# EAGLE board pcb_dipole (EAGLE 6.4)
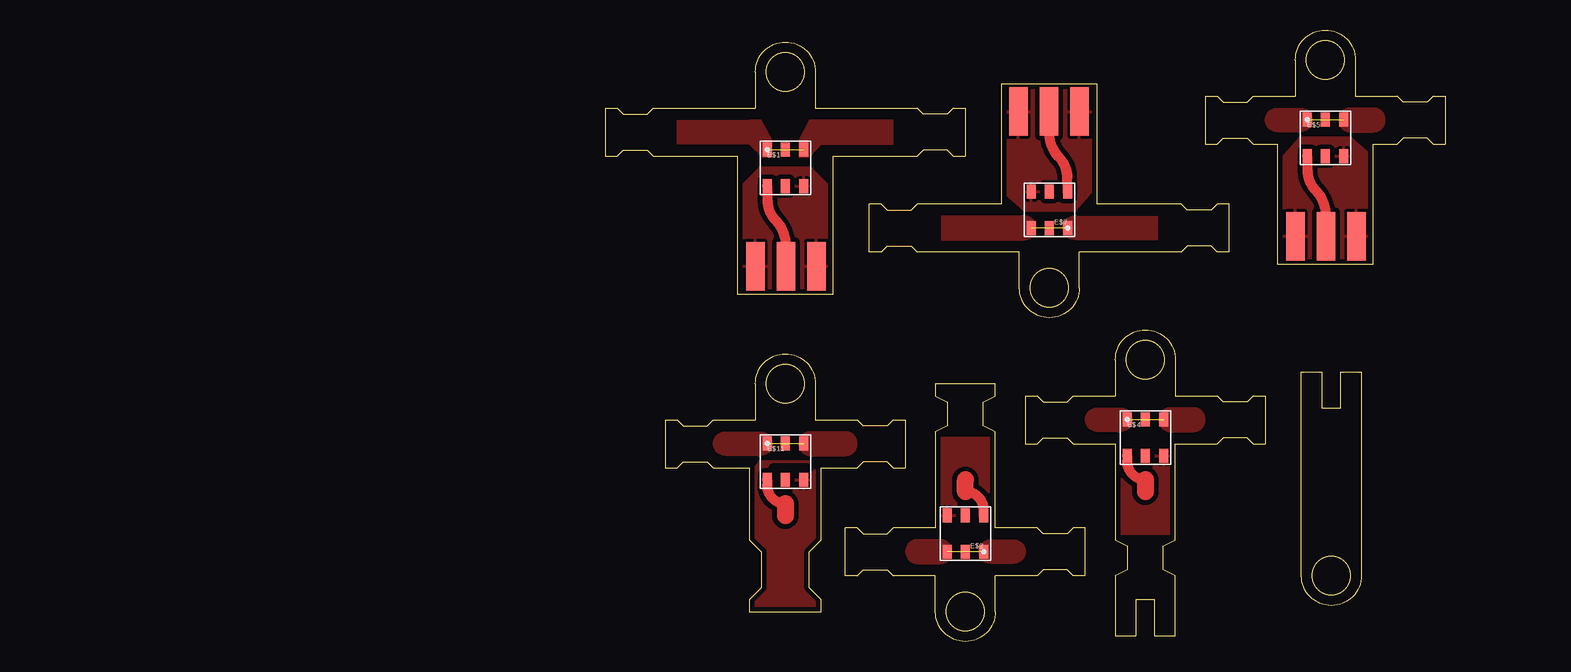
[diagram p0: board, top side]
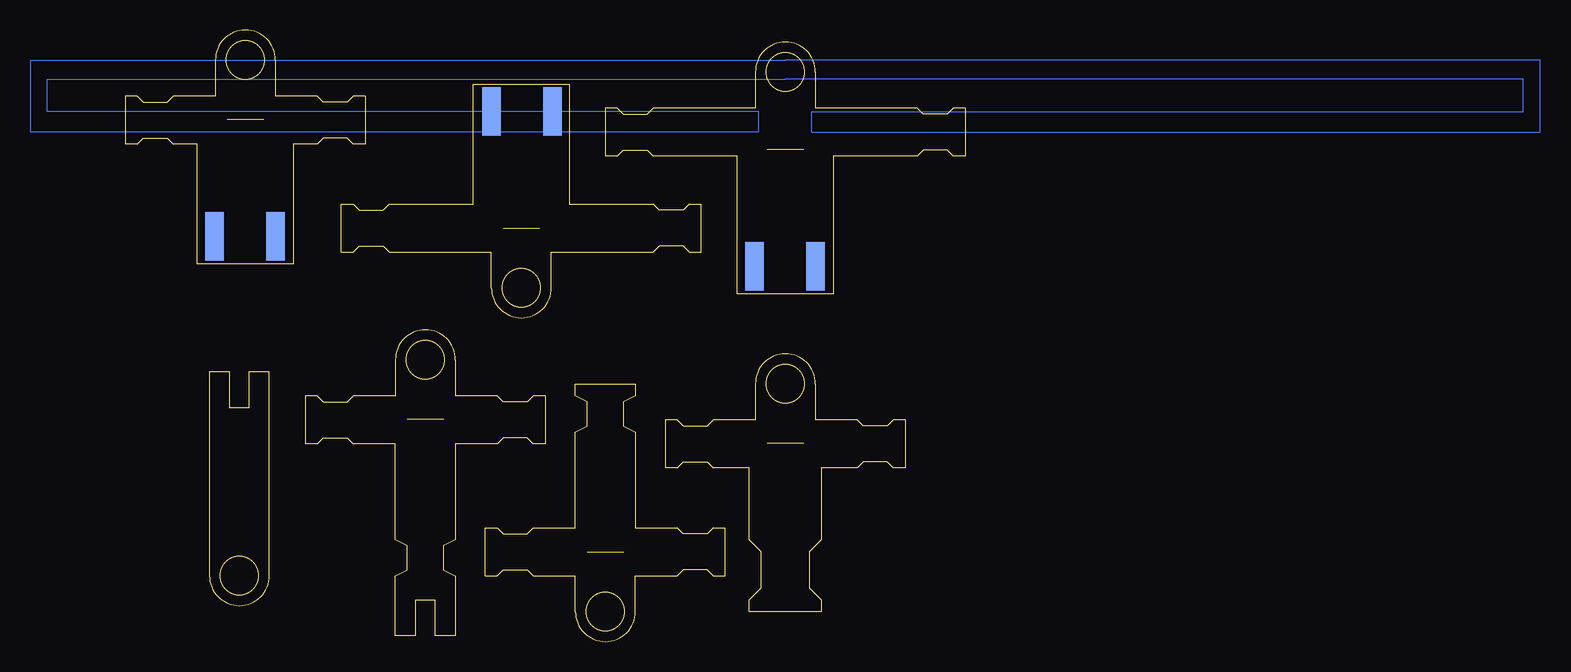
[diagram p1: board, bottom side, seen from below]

Size 70 x 51 mm. Coordinates in mm from the lower left corner, seen from the top.
Outline: 204 segments
Outline: circle at 15,47.5 radius 1.6
Outline: circle at 37,29.5 radius 1.6
Outline: circle at 15,21.5 radius 1.6
Outline: circle at 30,2.5 radius 1.6
Outline: circle at 45,23.5 radius 1.6
Outline: circle at 60.5,5.5 radius 1.6
Outline: circle at 60,48.5 radius 1.6
Copper layers (1*16): Top 0.035mm / dielectric 1.5mm / Bottom 0.035mm
Design rules "default *": minimum track width 10mil, minimum drill 24mil, track to track 8mil, track to pad 8mil, pad to pad 8mil, via to via 8mil, smd to smd 8mil, copper to edge 4mil, drill to drill 8mil, minimum pad ring 10mil, minimum via ring 8mil, stop-mask expansion 4mil, vias tented up to drill 0mil, thermal gap 10mil
tRestrict: 5 lines
bRestrict: 1 lines

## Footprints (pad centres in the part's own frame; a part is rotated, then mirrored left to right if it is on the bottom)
COILCRAFTWBC_SERIES = smd 0.76 x 1.14: P$1 -1.52,1.52; P$2 0,1.52; P$3 1.52,1.52; P$4 1.52,-1.52; P$5 0,-1.52; P$6 -1.52,-1.52
SMA-EDGE = smd 1.524 x 4.064: GND@0 0,0; GND@1 5.08,0; SIG 2.54,0 | smd 1.524 x 4.064 bottom: GND@2 0,0; GND@3 5.08,0

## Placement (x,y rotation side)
E$1  [COILCRAFTWBC_SERIES]  15,39.5 0 top
E$2  [COILCRAFTWBC_SERIES]  30,9 180 top
E$3  [SMA-EDGE]  12.5,31.3 0 top
E$4  [COILCRAFTWBC_SERIES]  45,17 0 top
E$5  [COILCRAFTWBC_SERIES]  60,42 0 top
E$6  [SMA-EDGE]  57.5,33.8 0 top
E$7  [COILCRAFTWBC_SERIES]  37,36 180 top
E$8  [SMA-EDGE]  39.5,44.2 180 top
E$11  [COILCRAFTWBC_SERIES]  15,15 0 top

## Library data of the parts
E$1 E$2 E$4 E$5 E$7 E$11 = RF components lasser
E$3 E$6 E$8 = SparkFun-Connectors

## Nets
FOL: E$1.P$1 E$1.P$3
FOL1: E$2.P$1 E$2.P$3
FOL2: E$4.P$1 E$4.P$3
FOL3: E$7.P$1 E$7.P$3
FOL4: E$5.P$1 E$5.P$3
FOL5: E$11.P$1 E$11.P$3
GND: E$1.P$4 E$3.GND@0 E$3.GND@1
GND1: E$2.P$4
GND2: E$4.P$4
GND4: E$5.P$4 E$6.GND@0 E$6.GND@1
GND5: E$7.P$4 E$8.GND@0 E$8.GND@1
GND6: E$11.P$4
S$3: E$2.P$6
S$5: E$1.P$6 E$3.SIG
S$7: E$4.P$6
S$8: E$7.P$6 E$8.SIG
S$9: E$5.P$6 E$6.SIG
S$11: E$11.P$6

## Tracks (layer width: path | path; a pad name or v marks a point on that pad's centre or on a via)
FOL  (1 unrouted)
  pour Top (no thermals): 12,41.5 13.1,40.4 13.9,40.4 13.9,41.8 13,43.5 12,43.5
  pour Top (no thermals): 16.1,40.4 17,40.4 18,41.5 18,43.5 17,43.5 16.1,41.8
FOL1  (1 unrouted)
  pour Top (no thermals): 35,7.5 arc-90 34,6.5 32.1,6.5 arc-90 31.1,7.5 arc-90 32.1,8.5 34,8.5 arc-90
  pour Top (no thermals): 27.9,8.5 26,8.5 arc90 25,7.5 arc90 26,6.5 27.9,6.5 arc90 28.9,7.5 arc90
FOL2  (1 unrouted)
  pour Top (no thermals): 40,18.5 arc-90 41,19.5 42.9,19.5 arc-90 43.9,18.5 arc-90 42.9,17.5 41,17.5 arc-90
  pour Top (no thermals): 47.1,17.5 49,17.5 arc90 50,18.5 arc90 49,19.5 47.1,19.5 arc90 46.1,18.5 arc90
FOL3  (1 unrouted)
  pour Top (no thermals): 46,33.5 39.1,33.5 arc-90 38.1,34.5 arc-90 39.1,35.5 46,35.5
  pour Top (no thermals): 28,33.5 34.9,33.5 arc90 35.9,34.5 arc90 34.9,35.5 28,35.5
FOL4  (1 unrouted)
  pour Top (no thermals): 55,43.5 arc-90 56,44.5 57.9,44.5 arc-90 58.9,43.5 arc-90 57.9,42.5 56,42.5 arc-90
  pour Top (no thermals): 62.1,42.5 64,42.5 arc90 65,43.5 arc90 64,44.5 62.1,44.5 arc90 61.1,43.5 arc90
FOL5  (1 unrouted)
  pour Top (no thermals): 9,16.5 arc-90 10,17.5 12.9,17.5 arc-90 13.9,16.5 arc-90 12.9,15.5 10,15.5 arc-90
  pour Top (no thermals): 17.1,15.5 20,15.5 arc90 21,16.5 arc90 20,17.5 17.1,17.5 arc90 16.1,16.5 arc90
GND
  pour Top (isolate 0.4): 9,26.5 21,26.5 21,35.59 17.09,39.5 12.88,39.5 9,35.62
GND1
  pour Top (isolate 0.4): 36,23.5 24,23.5 24,12.41 27.91,9 32.12,9 36,13.38
GND2
  pour Top (isolate 0.4): 39,2.5 51,2.5 51,13.59 47.09,17 42.88,17 39,12.62
GND3
  pour Bottom (isolate 0.4): 67,-31.5 55,-31.5 55,-22.41 58.91,-17 63.12,-17 67,-22.38
GND4
  pour Top (isolate 0.4): 54,27.5 66,27.5 66,38.59 62.09,42 57.88,42 54,37.62
GND5
  pour Top (isolate 0.4): 43,50.5 31,50.5 31,39.41 34.91,36 39.12,36 43,40.38
GND6
  pour Top (isolate 0.4): 9,0.5 21,0.5 21,11.59 17.09,15 12.88,15 9,10.62
S$1
  Bottom 0.05: 15,48.5 77.9,48.5 77.9,42.5 17.2,42.5 17.2,44.2 76.5,44.2 76.5,46.9 15,46.9
S$2
  Bottom 0.05: 15,48.5 -47.9,48.5 -47.9,42.5 12.8,42.5 12.8,44.2 -46.5,44.2 -46.5,46.9 15,46.9
S$3
  Top 0.813: E$2.P$6 31.52,10.98 arc90 30,12.5
  Top 1.422: 30,12.5 30,13.5
S$4
  pour Top: 18,41.5 24,41.5 24,43.5 18,43.5
S$5
  Top 0.813: E$1.P$6 13.5,36.8 arc43 14.2,35.1 arc-51 15,32.7 15.04,32.7 E$3.SIG
S$6
  pour Top: 12,41.5 6,41.5 6,43.5 12,43.5
S$7
  Top 0.813: E$4.P$6 43.48,15.02 arc90 45,13.5
  Top 1.422: 45,13.5 45,12.5
S$8
  Top 0.813: E$7.P$6 38.5,38.7 arc43 37.8,40.4 arc-51 37,42.8 36.96,42.8 E$8.SIG
S$9
  Top 0.813: E$5.P$6 58.5,39.3 arc43 59.2,37.6 arc-51 60,35.2 60.04,35.2 E$6.SIG
S$11
  Top 0.813: E$11.P$6 13.48,13.02 arc90 15,11.5
  Top 1.422: 15,11.5 15,10.5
